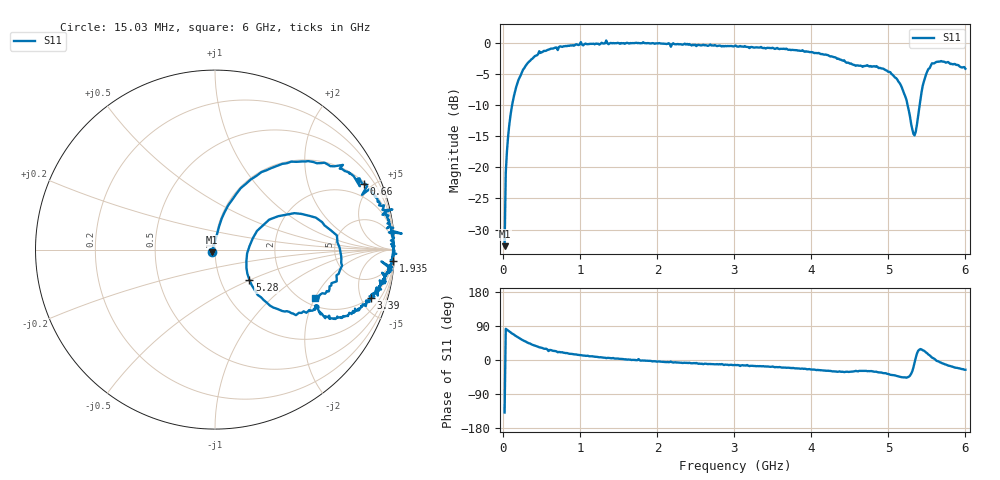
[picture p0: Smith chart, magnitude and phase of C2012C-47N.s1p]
!	Network	Analyzer	HP8753E.07.74:	Oct	30	2002	Serial	No.	JP38451487
!	Hewlett-Packard
!	7	Sep	2009	10:56:05
!	Frequency	S11
#	HZ	S	RI	R	50
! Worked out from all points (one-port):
!   400 points, 15.03 MHz to 6 GHz, reference 50 ohm
!   lowest |S11| = -32.7 dB at 15.03 MHz (marker M1), VSWR 1.05, Z = 48.3 - j1.49 ohm
!   |S11| at or under -10 dB: start of sweep to 113.1 MHz; 5.249 GHz to 5.405 GHz (156.7 MHz wide, 2.94 % of centre)
!   S11 on the Smith chart (normalised r, x): 15.03 MHz: 0.97, -0.03; 660 MHz: 1.10, +4.50; 1.935 GHz: 3, -31; 3.39 GHz: 1.95, -6.06; 5.28 GHz: 1.37, -0.50; 6 GHz: 2.31, -2.01
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1.502992e7  -0.0174 -0.0154
3.002985e7  0.0122 0.0894
4.502978e7  0.0233 0.131
9.002955e7  0.0737 0.247
1.500292e8  0.173 0.367
2.850286e8  0.425 0.49
4.650277e8  0.713 0.472
6.600267e8  0.83 0.365
7.650262e8  0.869 0.323
1.335023e9  1.04 0.0894
1.365023e9  0.969 0.0958
1.515022e9  0.98 0.0503
1.93502e9  0.992 -0.0632
2.265019e9  0.971 -0.111
3.015015e9  0.925 -0.222
3.390013e9  0.87 -0.267
3.765011e9  0.816 -0.315
4.515007e9  0.586 -0.348
4.845006e9  0.557 -0.334
5.025005e9  0.451 -0.365
5.160004e9  0.325 -0.323
5.265004e9  0.205 -0.199
5.280004e9  0.192 -0.17
5.340003e9  0.179 -0.0211
5.460003e9  0.442 0.203
5.565002e9  0.679 0.079
5.625002e9  0.702 -0.0281
6e9  0.558 -0.268
